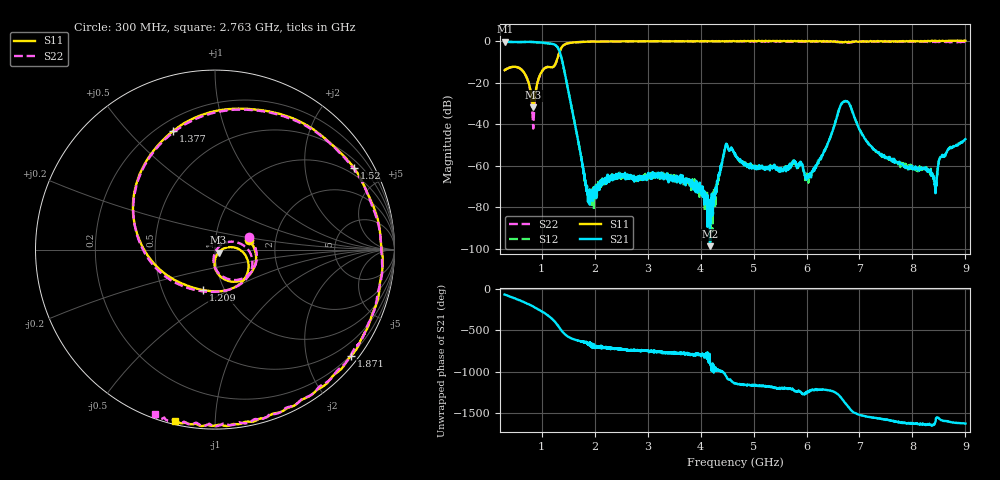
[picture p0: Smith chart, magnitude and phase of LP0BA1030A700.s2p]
!Agilent Technologies,E8358A,US41080443,A.07.50.56
!Agilent E8358A: A.07.50.56
!Date: Wednesday, March 04, 2015 10:21:57
!Correction: S11(Full 2 Port(1,2))
!S21(Full 2 Port(1,2))
!S12(Full 2 Port(1,2))
!S22(Full 2 Port(1,2))
!S2P File: Measurements: S11, S21, S12, S22:Log Frequency Sweep
# Hz S  dB  R 50
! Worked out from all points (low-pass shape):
!   3201 points, 300 MHz to 9 GHz, reference 50 ohm
!   highest |S21| = -0.33 dB at 300.6 MHz (marker M1); lowest = -98.7 dB at 4.178 GHz (marker M2)
!   |S21| within 3 dB of the highest: start of sweep to 1.308 GHz
!   lowest |S11| = -31.9 dB at 840.3 MHz (marker M3), VSWR 1.05, Z = 52 - j1.68 ohm
!   |S11| at or under -10 dB: start of sweep to 1.275 GHz
!   |S22| runs from -42.1 to 0.0 dB; largest |S21 - S12| = 0.0064
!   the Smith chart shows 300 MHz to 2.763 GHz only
!   S11 on the Smith chart (normalised r, x): 300 MHz: 1.46, +0.16; 1.209 GHz: 0.80, -0.38; 1.377 GHz: 0.26, +0.68; 1.52 GHz: 0.74, +3.53; 1.871 GHz: 0.18, -2.90; 2.763 GHz: 0.02, -0.79
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3e8  -14.03 15.4  -0.33 -70.9  -0.38 -71.0  -14.02 19.9
3.006384e8  -14.03 15.2  -0.33 -71.1  -0.38 -71.2  -13.99 19.7
6.909992e8  -16.17 -77.9  -0.44 -169.9  -0.49 -169.9  -16.15 -74.1
8.402568e8  -31.89 -39.5  -0.45 144.2  -0.49 144.1  -42.14 -30.6
9.061199e8  -21.50 9.6  -0.54 121.8  -0.58 121.7  -21.86 31.0
1.030479e9  -13.71 -25.1  -0.86 74.9  -0.90 74.8  -13.71 -10.2
1.208591e9  -12.57 -106.4  -1.45 -11.9  -1.50 -11.9  -12.54 -92.8
1.293665e9  -8.64 -173.2  -2.78 -74.0  -2.82 -74.0  -8.80 -168.5
1.377388e9  -3.08 109.4  -8.50 -148.1  -8.55 -148.3  -3.12 108.4
1.520495e9  -0.93 30.5  -26.20 133.2  -26.25 133.2  -0.93 27.5
1.75137e9  -0.48 -22.6  -56.83 83.9  -56.53 84.5  -0.45 -26.4
1.87067e9  -0.33 -37.9  -72.20 55.1  -72.01 59.0  -0.35 -43.1
2.76315e9  -0.18 -103.2  -66.84 -18.7  -66.61 -29.0  -0.21 -109.9
3.203074e9  -0.09 -122.6  -63.37 -40.6  -65.15 -39.1  -0.08 -126.8
4.177986e9  -0.19 -154.1  -98.73 -175.5  -79.16 -155.9  -0.10 -152.0
4.472079e9  -0.10 -161.5  -50.26 36.4  -50.20 35.4  -0.21 -157.0
4.651453e9  -0.16 -165.7  -54.11 -63.1  -54.56 -60.9  -0.07 -160.8
6.106022e9  -0.07 163.3  -62.50 -145.0  -63.35 -143.9  -0.29 176.1
6.726111e9  -0.40 153.7  -28.90 64.2  -29.08 64.3  -0.73 164.4
7.552286e9  -0.14 139.4  -55.83 -146.5  -57.12 -145.1  -0.27 147.4
8.336952e9  -0.09 125.6  -62.71 157.7  -64.38 165.4  -0.37 123.8
9e9  0.12 114.1  -47.23 172.0  -47.36 172.6  -0.33 108.9
